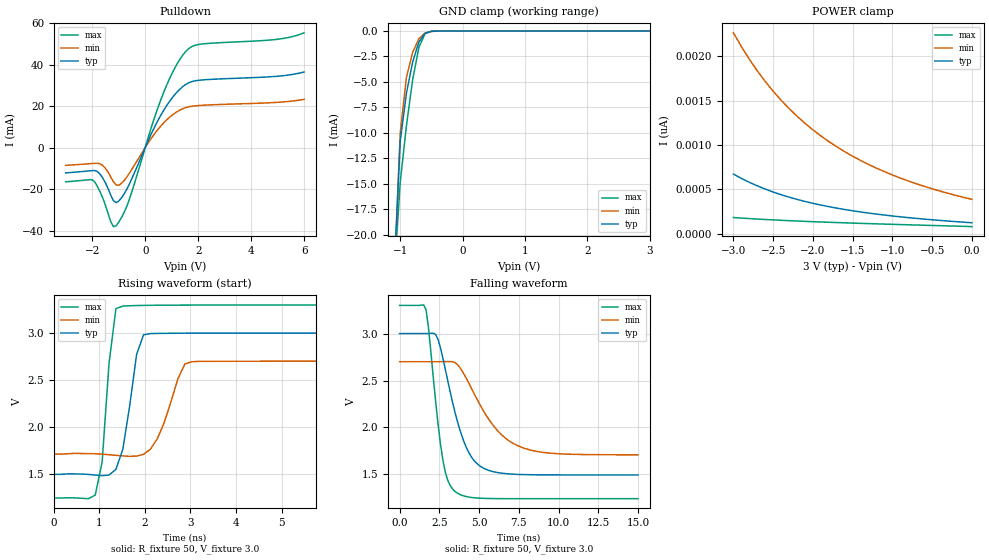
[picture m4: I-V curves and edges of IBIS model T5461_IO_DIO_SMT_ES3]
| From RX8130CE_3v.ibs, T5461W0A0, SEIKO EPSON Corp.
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[Model]   T5461_IO_DIO_SMT_ES3
Model_type I/O_open_drain
Enable Active-High
Polarity Non-Inverting
Vinh=2.64
Vinl=0.54
Vmeas=1.50
Vref=3.3
Rref=5000
C_comp   2.5p   2.0p   3.0p
[Temperature Range] 25   85   -40
[Voltage Range]   3.0   2.7   3.3
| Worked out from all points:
|   slope of the pulldown table from 0 to 0.45 V, typ, clamps not added: 36.5 ohm
|   GND clamp passes 1 mA (typ) near -0.69 V on its own axis
|   falling waveform, R_fixture 50, V_fixture 3.0: 20-80 % time 1.41ns typ, 2.25ns min, 804ps max; typ from 3 V to 1.49 V
|   rising waveform, R_fixture 50, V_fixture 3.0: 20-80 % time 271ps typ, 416ps min, 202ps max; typ from 1.49 V to 3 V
[Pulldown]
-3V       -12.19mA   -8.567mA   -16.5mA
-2V       -11.1mA    -7.676mA   -15.51mA
-1.6V     -14.7mA    -8.655mA   -24.32mA
-1.3V     -22.98mA   -14.16mA   -35.77mA
-1.1V     -26.54mA   -17.92mA   -37.73mA
-600mV    -17.64mA   -12.42mA   -25.02mA
300mV     8.527mA    5.742mA    12.5mA
700mV     18.02mA    11.94mA    26.7mA
1.2V      26.75mA    17.29mA    40.29mA
1.6V      30.98mA    19.54mA    47.25mA
2.1V      32.57mA    20.37mA    49.89mA
6V        36.47mA    23.28mA    55.36mA
[GND Clamp]
-3V       -502.2mA   -418.5mA   -628.9mA
-1.1V     -24.07mA   -25.42mA   -24.54mA
-1V       -10.87mA   -10.09mA   -14.91mA
-900mV    -6.13mA    -4.561mA   -9.309mA
-800mV    -3.058mA   -2.097mA   -4.786mA
-700mV    -1.078mA   -757.4uA   -1.604mA
-600mV    -224.6uA   -189.6uA   -244.1uA
-500mV    -33.81uA   -37.1uA    -22.82uA
-400mV    -4.624uA   -6.222uA   -2.07uA
3V        124.1pA    455.9pA    73.37pA
[POWER Clamp]
-3V       672pA      2.262nA    183.3pA
-2.8V     579.6pA    1.965nA    171.4pA
-2.7V     539.7pA    1.834nA    166pA
-2.5V     470.3pA    1.605nA    156.4pA
-2.4V     440.2pA    1.503nA    152pA
-2.2V     387.4pA    1.324nA    143.9pA
-2V       343.1pA    1.17nA     136.5pA
-1.8V     305.5pA    1.039nA    129.8pA
-1.4V     245.9pA    825.7pA    117.6pA
-1V       200.8pA    662.6pA    106.6pA
-500mV    157.9pA    507.1pA    93.84pA
0V        124.1pA    388pA      81.19pA
[Falling Waveform]
R_fixture=50
V_fixture=3.0
V_fixture_min=2.7
V_fixture_max=3.3
0s        3V         2.7V       3.3V
1.667ns   3V         2.7V       3.252V
2.273ns   2.989V     2.7V       2.268V
2.727ns   2.736V     2.701V     1.648V
3.03ns    2.497V     2.702V     1.437V
3.485ns   2.161V     2.691V     1.318V
4.697ns   1.644V     2.358V     1.25V
5.909ns   1.528V     2.018V     1.242V
7.273ns   1.501V     1.819V     1.241V
15ns      1.493V     1.708V     1.241V
[Rising Waveform]
R_fixture=50
V_fixture=3.0
V_fixture_min=2.7
V_fixture_max=3.3
0s        1.493V     1.708V     1.241V
909.1ps   1.486V     1.713V     1.272V
1.061ns   1.479V     1.709V     1.622V
1.212ns   1.486V     1.703V     2.676V
1.364ns   1.547V     1.696V     3.261V
1.515ns   1.761V     1.69V      3.287V
1.818ns   2.773V     1.688V     3.293V
1.97ns    2.981V     1.707V     3.295V
3.03ns    2.999V     2.694V     3.298V
15ns      3V         2.7V       3.3V
[Ramp]
R_load=50
dV/dt_r   9.040E-1/2.637E-10   5.950E-1/4.090E-10   1.236E+0/1.781E-10
dV/dt_f   9.040E-1/1.402E-9   5.949E-1/2.252E-9   1.235E+0/8.012E-10
|[End   T5461_IO_DIO_SMT_ES3
